FUNCTION_BLOCK FB_LN_IED_LD1_LEDGGIO5 EXTENDS FB_AcsiCommonLogicalNodeClass
VAR_INPUT
	NamPlt: FB_DO_IED_LD1_LEDGGIO5_NamPlt := (sClass:='LPL', bLinkResult:=THIS^.AddDataToContainer(ipData:=NamPlt));
	Beh: FB_DO_IED_LD1_LEDGGIO5_Beh := (sClass:='ENS', bLinkResult:=THIS^.AddDataToContainer(ipData:=Beh));
	Health: FB_DO_IED_LD1_LEDGGIO5_Health := (sClass:='ENS', bLinkResult:=THIS^.AddDataToContainer(ipData:=Health));
	Mod_: FB_DO_IED_LD1_LEDGGIO5_Mod := (sObjectName:='Mod', sClass:='ENC', bLinkResult:=THIS^.AddDataToContainer(ipData:=Mod_));
	AnOut1: FB_DO_IED_LD1_LEDGGIO5_AnOut1 := (sClass:='APC', bLinkResult:=THIS^.AddDataToContainer(ipData:=AnOut1));
	SPCSO1: FB_DO_IED_LD1_LEDGGIO5_SPCSO1 := (sClass:='SPC', bLinkResult:=THIS^.AddDataToContainer(ipData:=SPCSO1));
	DPCSO1: FB_DO_IED_LD1_LEDGGIO5_DPCSO1 := (sClass:='DPC', bLinkResult:=THIS^.AddDataToContainer(ipData:=DPCSO1));
	ISCSO1: FB_DO_IED_LD1_LEDGGIO5_ISCSO1 := (sClass:='INC', bLinkResult:=THIS^.AddDataToContainer(ipData:=ISCSO1));
END_VAR
VAR
END_VAR

END_FUNCTION_BLOCK
